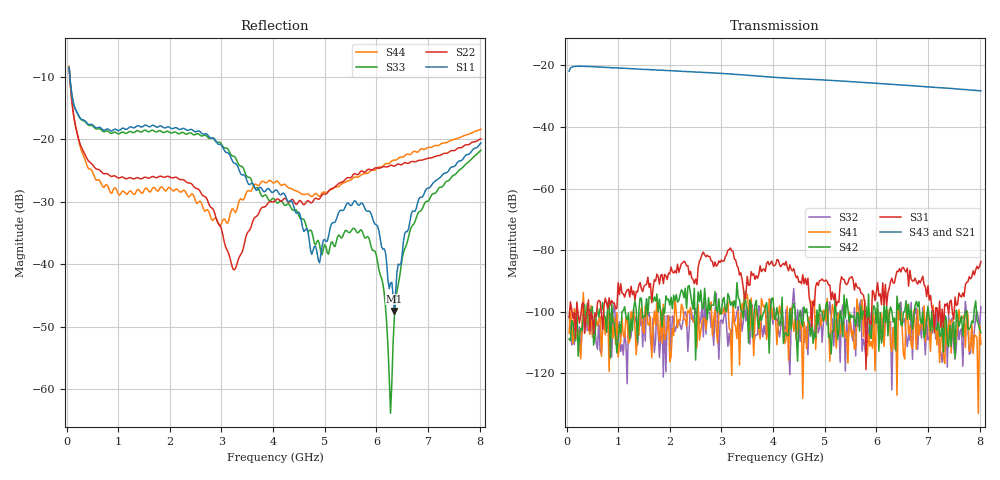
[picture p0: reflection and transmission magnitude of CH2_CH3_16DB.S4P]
!Agilent Technologies,E5071C,MY46316741,A.11.02
!Date: Thu May 28 14:40:48 2026
!Data & Calibration Information:
!1:CH2 INPUT 2:CH2 OUTPUT 3:CH3 INPUT 4:CH3 OUTPUT
!Freq	S11:SOLT4(ON)	S12:SOLT4(ON)	S13:SOLT4(ON)	S14:SOLT4(ON)
!	S21:SOLT4(ON)	S22:SOLT4(ON)	S23:SOLT4(ON)	S24:SOLT4(ON)
!	S31:SOLT4(ON)	S32:SOLT4(ON)	S33:SOLT4(ON)	S34:SOLT4(ON)
!	S41:SOLT4(ON)	S42:SOLT4(ON)	S43:SOLT4(ON)	S44:SOLT4(ON)
!PortZ  Port1:50+j0  Port2:50+j0  Port3:50+j0  Port4:50+j0
!Above PortZ is port z conversion or system Z0 setting when saving the data.
!When reading, reference impedance value at option line is always used.
# Hz S dB R 50
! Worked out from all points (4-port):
!   320 points, 50 MHz to 8.025 GHz, reference 50 ohm
!   strongest paths, dB at 50 MHz, 2.05 GHz, 4.05 GHz, 6.05 GHz, 8.025 GHz:
!     S43: -21.9, -21.7, -23.9, -25.8, -28.2
!     S21: -21.9, -21.8, -24.1, -26.1, -28.4
!     S31: -101.8, -87.0, -84.6, -94.9, -83.7
!     S42: -108.8, -99.1, -102.3, -112.8, -106.8
!     S41: -107.0, -105.3, -102.8, -103.1, -110.5
!     S32: -101.7, -101.3, -102.7, -108.5, -98.4
!   lowest |S11| = -47.5 dB at 6.35 GHz (marker M1), VSWR 1.01, Z = 49.6 - j0.193 ohm
!   |S11| at or under -10 dB: 64.67 MHz to end of sweep
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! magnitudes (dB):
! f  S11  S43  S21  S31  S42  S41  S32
! 50 MHz  -8.5  -21.9  -21.9  -101.8  -108.8  -107.0  -101.7
! 700 MHz  -18.5  -20.6  -20.7  -105.7  -97.0  -105.5  -104.4
! 3.25 GHz  -23.8  -22.9  -23.0  -82.9  -96.4  -103.6  -103.6
! 5.85 GHz  -31.5  -25.6  -25.8  -101.8  -94.3  -107.3  -109.3
! 6.275 GHz  -43.0  -26.1  -26.3  -90.3  -98.4  -110.9  -103.3
! 6.35 GHz  -47.5  -26.2  -26.4  -90.7  -102.0  -112.0  -109.7
! 8.025 GHz  -20.6  -28.2  -28.4  -83.7  -106.8  -110.5  -98.4
